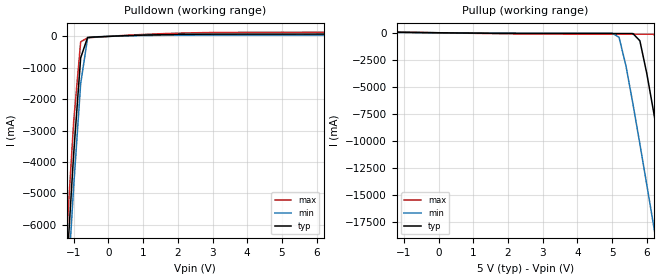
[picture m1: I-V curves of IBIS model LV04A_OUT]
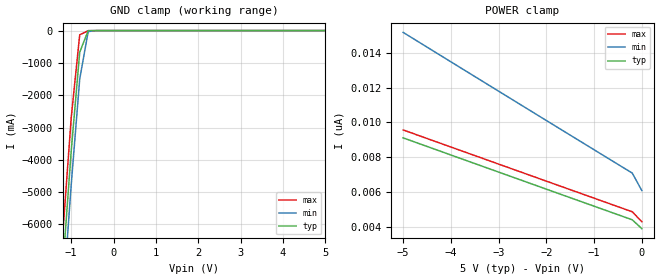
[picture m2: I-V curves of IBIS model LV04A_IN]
|   TEXAS INSTRUMENTS INCORPORATED
|   Advanced Bus Interface Group
|   IBIS Model of LV04A (Vcc=5V)
|   CMOS Hex Inverter
|   SOIC 14-pin (D) Package
[IBIS Ver]   1.1
[File Name]   lv04a_5.ibs
[File Rev]   2.0
[Date]   9/6/97
[Source]   File originated at Texas Instruments, Inc.
[Notes]   The following is an IBIS list for the LV04A.
|   - All test data contained in this file are derived from
|   hspice(tm) simulations.
|   - File created by Teruo Ishii, SLL Applications.
[Disclaimer] Property of Texas Instruments Incorporated.  Unauthorized
   reproduction and/or distribution is strictly prohibited.
   This product is protected under copyright law.
   Created 1997, (C) Copyright 1997, Texas Instruments Inc.,
   All Rights Reserved
   UNLESS THERE IS A SIGNED, WRITTEN AGREEMENT TO THE
   CONTRARY, TEXAS INSTRUMENTS ("TI") IS PROVIDING THE IBIS
   MODELS "AS IS" AND WITHOUT ANY WARRANTY, EXPRESSED OR
   IMPLIED.  TI assumes no liability for:
   1) the accuracy of the IBIS models provided to your
   company;
   2) the proper functioning of these IBIS models in your
   design or for any resulting applications; or
   3) infringement of patents, copyrights or intellectual
   property rights resulting from your use of these IBIS
   models.
   TI provides IBIS Models as a service to our customers.
   You and your company shall not distribute, sell or give
   these models to anyone else without prior written
   permission from TI.
   TI reserves the right to make changes to our products or
   to discontinue any semiconductor product or service
   without notice, and advises our customers to obtain the
   latest version of relevant information to verify, before
   placing orders, that the information being relied on is
   current.
   Please be aware that your receipt and use of the IBIS
   information provided shall serve as acceptance of these
   terms and conditions.  If you do not accept these terms,
   you should return or destroy the IBIS models and any
   other accompanying information immediately.
[Component]   LV04A(Hex_Inverter)
[Manufacturer]  Texas Instruments
[Package]
|   typ   min   max
R_pkg   0.020   0.018   0.021
L_pkg   3.17nH   2.22nH   4.32nH
C_pkg   0.35pF   0.20pF   0.50pF
[Pin]   signal_name   model_name   R_pin   L_pin   C_pin
1   1A   LV04A_IN   0.018   4.30nH   0.50pF
2   1Y   LV04A_OUT   0.021   3.39nH   0.43pF
3   2A   LV04A_IN   0.019   2.24nH   0.26pF
4   2Y   LV04A_OUT   0.020   2.27nH   0.21pF
5   3A   LV04A_IN   0.020   2.22nH   0.20pF
6   3Y   LV04A_OUT   0.021   3.43nH   0.38pF
7   GND   GND   0.020   4.32nH   0.50pF
8   4Y   LV04A_OUT   0.020   4.32nH   0.50pF
9   4A   LV04A_IN   0.021   3.43nH   0.38pF
10   5Y   LV04A_OUT   0.020   2.22nH   0.20pF
11   5A   LV04A_IN   0.020   2.27nH   0.21pF
12   6Y   LV04A_OUT   0.019   2.24nH   0.26pF
13   6A   LV04A_IN   0.021   3.39nH   0.43pF
14   VCC   POWER   0.018   4.30nH   0.50pF
| Models and submodels in the file (2): LV04A_OUT (Output), LV04A_IN (Input)
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|   Model LV04A_OUT
[Model]   LV04A_OUT
Model_type   Output
Polarity   Inverting
|variable   typ   min   max
C_comp   4.0pF   NA   NA
[Voltage range]   5.0   4.5   5.5
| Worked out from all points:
|   slope of the pulldown table from 0 to 0.75 V, typ, clamps not added: 23.2 ohm
|   slope of the pullup table from 0 to 0.75 V, typ, clamps not added: 29.3 ohm
[Pulldown]
|   Voltage   I(typ)   I(min)   I(max)
-5V       -81.99A    -82.92A    -81.08A
-1.2V     -7.334A    -8.394A    -6.29A
-1V       -3.716A    -4.76A     -2.696A
-800mV    -684.6mA   -1.507A    -174.2mA
-600mV    -32.04mA   -49.56mA   -44.95mA
-400mV    -20.26mA   -14.47mA   -29.3mA
400mV     18.84mA    13.27mA    27.19mA
2.4V      67.49mA    39.34mA    113mA
6.8V      78.71mA    45.01mA    135.4mA
10V       118.3mA    69.61mA    192.4mA
[Pullup]   | Note: Vtable = Vcc - Voutput
|   Voltage   I(typ)   I(min)   I(max)
-5V       65.33mA    38.18mA    202.7mA
5V        -72.3mA    -39.77mA   -130.3mA
5.2V      -72.34mA   -419.6mA   -130.3mA
5.4V      -72.64mA   -3.083A    -130.4mA
5.6V      -75.89mA   -6.59A     -130.4mA
5.8V      -740.7mA   -10.3A     -130.8mA
6.2V      -7.404A    -17.94A    -139.2mA
6.4V      -11.17A    -21.82A    -1.238A
6.8V      -18.88A    -29.62A    -8.294A
7.2V      -26.69A    -37.47A    -15.98A
7.4V      -30.61A    -41.4A     -19.88A
10V       -82.06A    -92.89A    -71.28A
[Ramp]
|Variable   typ   min   max
dV/dt_r   1.7549E+00/1.3582E-09  1.1040E+00/2.2255E-09  2.3393E+00/6.7797E-10
dV/dt_f   1.8615E+00/1.6117E-09  1.1972E+00/2.4249E-09  2.4586E+00/1.0155E-09
|   Model LV04A_IN
[Model]   LV04A_IN
Model_type   Input
Polarity   Inverting
Vinl = 3.5V
Vinh = 1.5V
|variable   typ   min   max
C_comp   2.3pF   NA   NA
[Voltage Range]   5.0   4.5   5.5
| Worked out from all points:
|   GND clamp passes 1 mA (typ) near -0.46 V on its own axis
[GND_Clamp]
|   Voltage   I(typ)   I(min)   I(max)
-5V       -82A       -82.93A    -81.1A
-1.2V     -7.333A    -8.394A    -6.288A
-1V       -3.712A    -4.759A    -2.688A
-800mV    -668.4mA   -1.501A    -130.8mA
-600mV    -3.037mA   -30.13mA   -3.193mA
-400mV    -173.2uA   -104.7uA   -839.2uA
5V        3.916nA    7.599nA    3.537nA
[POWER_Clamp]   | Note: Vtable = Vcc - Voutput
|   Voltage   I(typ)   I(min)   I(max)
-5V       9.116nA    15.16nA    9.57nA
-2.4V     6.569nA    10.78nA    7.027nA
-200mV    4.423nA    7.098nA    4.883nA
0V        3.916nA    6.098nA    4.314nA
